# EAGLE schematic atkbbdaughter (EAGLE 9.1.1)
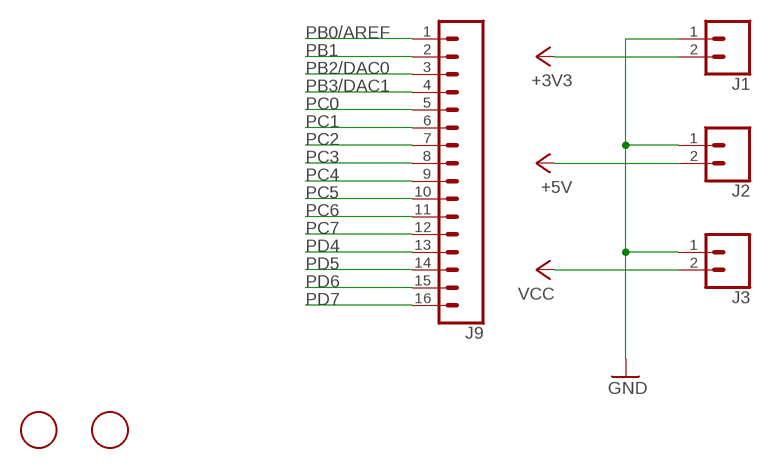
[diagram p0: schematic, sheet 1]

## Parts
J1  CONN_021X02_NO_SILK  [1X02_NO_SILK]
J2  CONN_021X02_NO_SILK  [1X02_NO_SILK]
J3  CONN_021X02_NO_SILK  [1X02_NO_SILK]
J4  FIDUCIALRCT  [FIDUCIAL_RECT_1MM]
J5  FIDUCIALRCT  [FIDUCIAL_RECT_1MM]
J9  CONN_161X16_NO_SILK  [1X16_NO_SILK]

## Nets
+3V3: J1.2
+5V: J2.2
GND: J1.1 J2.1 J3.1
PB0/AREF: J9.1
PB1: J9.2
PB2/DAC0: J9.3
PB3/DAC1: J9.4
PC0: J9.5
PC1: J9.6
PC2: J9.7
PC3: J9.8
PC4: J9.9
PC5: J9.10
PC6: J9.11
PC7: J9.12
PD4: J9.13
PD5: J9.14
PD6: J9.15
PD7: J9.16
VCC: J3.2

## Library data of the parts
J1-J3 = SparkFun-Connectors:CONN_02: Multi connection point. Often used as Generic Header-pin footprint for 0.1 inch spaced/style header connections
J4 J5 = connector:FIDUCIAL: For use by pick and place machines to calibrate the vision/machine, 1mm
J9 = SparkFun-Connectors:CONN_16: Multi connection point. Often used as Generic Header-pin footprint for 0.1 inch spaced/style header connections On any of the 0.1 inch spaced packages, you can populate with these: Break Away Headers - Straight (PRT-00116) Break Away Male Headers - Right Angle (PRT-00553) Female Headers (PRT-00115)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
